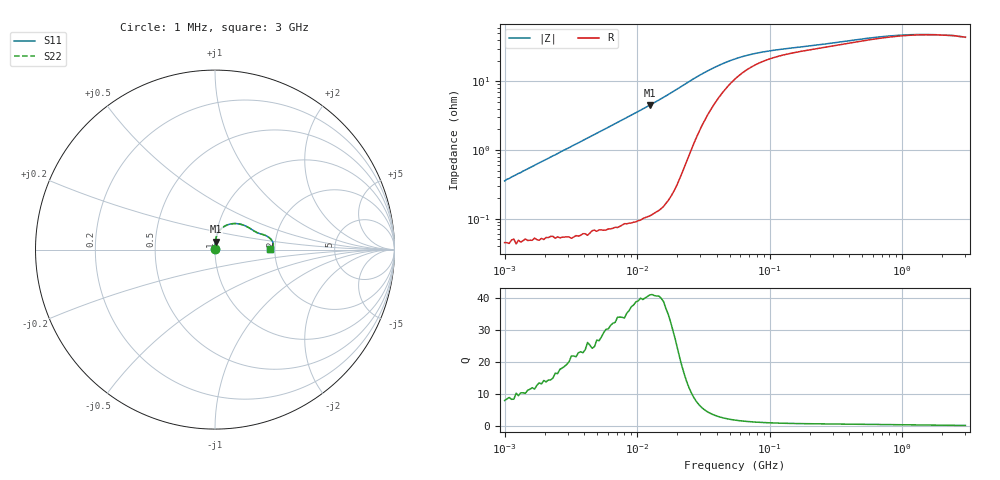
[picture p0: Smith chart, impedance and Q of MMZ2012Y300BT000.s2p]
! S-parameter Generated by TDK Corporation
! Copyright(C) 2016 TDK Corporation.
! All Rights Reserved.
! TDK P/N: MMZ2012Y300BT000 (Chip Beads)
! Property: |Z|=30¶ at 100MHz
! Size(LxWxT): 2x1.25x0.85mm, 0.079x0.049x0.033inches
! Model Type: s2p (Touchstone File Format Version 1.0)
! Frequency: DC=Yes Start=1MHz Stop=3000MHz 202points Log-sweep
! Note: This model was converted from impedance.
! Model Generated on May. 16, 2016
! Hash(MD5):
! Port Assignments:
!  1 ---@@@--- 2
! Applicable Conditions:
!  Temperature = 25 degC
!  DC Bias Current = 0 A
!  Small Signal Operation
! Terms and conditions regarding TDK Simulation Models
! (1)This simulation model is being provided solely for informational purposes. Please refer to the specifications of the products in terms of detailed characteristics of such products.
! (2)In no event shall TDK Corporation of any of its subsidiaries be liable for any loss or damage arising, directly or indirectly,
!  From any information contained in this simulation model, including, but not limited to loss or damages arising from any inaccuracies, omissions or errors in connection with such information.
! (3)Any and all copyrights on this simulation model are owned by TDK Corporation.
!  Duplication or redistribution of this simulation model without prior written permission from TDK Corporation is prohibited.
! (4)This simulation model is subject to any modification or change without any prior notice.
! (5)Neither TDK Corporation nor any of its subsidiaries shall make any warranty, express or implied,
!  Including but not limited to the correctness, implied warranties of merchantability and fitness for a particular purpose with respect to this simulation models.
! (6)The use of this simulation model shall be deemed to have consented to the terms and conditions hereof.
# MHz S MA R 50
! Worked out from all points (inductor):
!   201 points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, 1 MHz to 3 GHz, reference 50 ohm
!   read as one part in series: L = 56.5 nH near 1.041 MHz
!   highest Q = 40.7 at 12.45 MHz (marker M1), where L = 57.4 nH
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1  0.003539 82.5  0.9995 -0.2  0.9995 -0.2  0.003539 82.5
1.040844  0.00374 82.9  0.9995 -0.2  0.9995 -0.2  0.00374 82.9
1.323425  0.004686 84.2  0.9995 -0.3  0.9995 -0.3  0.004686 84.2
3.900413  0.01378 86.7  0.9993 -0.8  0.9993 -0.8  0.01378 86.7
7.400828  0.02618 86.8  0.9989 -1.5  0.9989 -1.5  0.02618 86.8
12.45355  0.04486 86.0  0.9979 -2.6  0.9979 -2.6  0.04486 86.0
14.61624  0.05336 85.5  0.9973 -3.1  0.9973 -3.1  0.05336 85.5
22.70269  0.08897 81.3  0.9905 -5.1  0.9905 -5.1  0.08897 81.3
26.64524  0.1069 77.5  0.9824 -6.1  0.9824 -6.1  0.1069 77.5
31.27247  0.1261 72.3  0.9692 -7.1  0.9692 -7.1  0.1261 72.3
41.38676  0.1596 61.4  0.9342 -8.6  0.9342 -8.6  0.1596 61.4
54.77226  0.1889 50.0  0.8905 -9.4  0.8905 -9.4  0.1889 50.0
66.90963  0.2049 42.7  0.8608 -9.3  0.8608 -9.3  0.2049 42.7
88.54986  0.2212 34.6  0.8276 -8.7  0.8276 -8.7  0.2212 34.6
121.9755  0.2346 28.0  0.8004 -7.9  0.8004 -7.9  0.2346 28.0
213.6344  0.2556 21.3  0.7675 -6.9  0.7675 -6.9  0.2556 21.3
457.0858  0.2926 15.6  0.7225 -6.3  0.7225 -6.3  0.2926 15.6
800.5644  0.3165 10.6  0.6914 -4.8  0.6914 -4.8  0.3165 10.6
1147.801  0.3245 7.4  0.6795 -3.5  0.6795 -3.5  0.3245 7.4
1645.649  0.3249 4.5  0.6766 -2.2  0.6766 -2.2  0.3249 4.5
2455.801  0.3167 1.8  0.6835 -0.8  0.6835 -0.8  0.3167 1.8
3000  0.305 0.7  0.6951 -0.3  0.6951 -0.3  0.305 0.7
